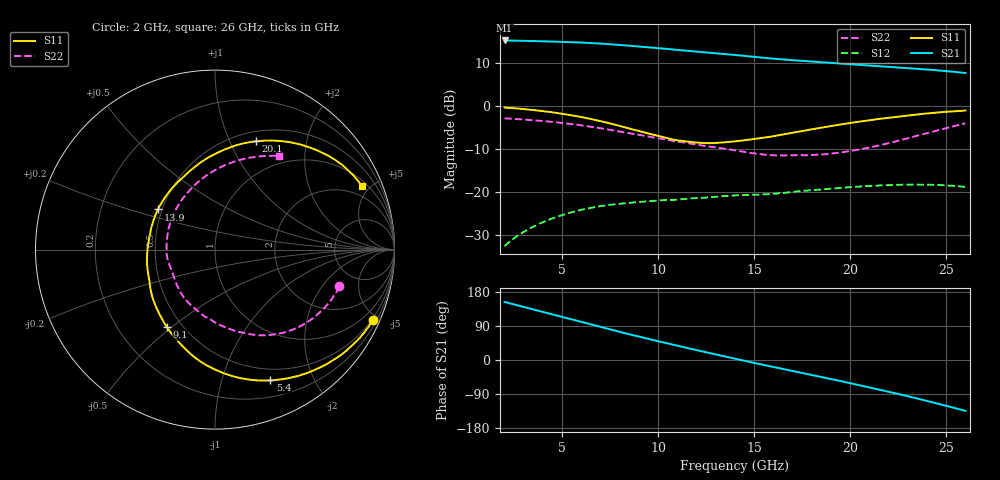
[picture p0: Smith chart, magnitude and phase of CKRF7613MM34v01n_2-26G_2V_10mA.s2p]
! CHUO DENSHI KOGYO Co.,Ltd.
! 26. October 2020
! CKRF7613MM34_RT5880
! N-channel HJ-FET
! Vds = 2 V, Id = 10 mA
# Hz S  MA  R 50
!	f	S11	S21	S12	S22
!	Hz	MAG	ANG	MAG	ANG	MAG	ANG	MAG	ANG
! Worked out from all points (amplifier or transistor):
!   241 points, 2 GHz to 26 GHz, reference 50 ohm
!   highest |S21| = 15.3 dB at 2 GHz (marker M1)
!   |S21| within 3 dB of that: start of sweep to 13.09 GHz
!   unconditionally stable (mu >= 1): 10.36 GHz to 18.29 GHz
!   at 6 GHz: K = 0.58, MSG = 19.4 dB, |S12| = -24.1 dB
!   at 14 GHz: K = 1.12, MAG = 14.2 dB, |S12| = -20.7 dB
!   at 26 GHz: K = 0.34, MSG = 13.3 dB, |S12| = -18.8 dB
!   lowest NFmin = 0.33 dB at 10 GHz
!   S11 on the Smith chart (normalised r, x): 2 GHz: 0.41, -4.64; 5.4 GHz: 0.37, -1.45; 9.1 GHz: 0.41, -0.48; 13.9 GHz: 0.47, +0.25; 20.1 GHz: 0.61, +1.25; 26 GHz: 1.29, +4.45
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2e9  0.9649 -24.1  5.826 153.1  0.02358 73.4  0.7222 -16.5
2.9e9  0.9316 -35.1  5.776 141.3  0.03353 66.7  0.7039 -24.0
3.8e9  0.8884 -46.3  5.713 129.4  0.04299 59.9  0.6787 -31.4
4.6e9  0.8436 -56.4  5.644 118.9  0.05058 54.0  0.6532 -38.2
5.4e9  0.7914 -67.0  5.57 108.4  0.05767 48.0  0.625 -45.1
6e9  0.7492 -75.2  5.504 100.5  0.06252 43.5  0.6002 -50.4
6.7e9  0.695 -85.1  5.405 91.2  0.06715 38.4  0.569 -56.6
7.4e9  0.6394 -95.4  5.29 82.0  0.07109 33.6  0.537 -62.8
8.2e9  0.5728 -107.6  5.119 71.6  0.07417 28.6  0.4986 -69.6
9.1e9  0.5075 -121.9  4.928 60.4  0.07738 24.0  0.46 -77.4
1e10  0.4521 -137.7  4.743 49.5  0.08006 19.9  0.4253 -85.3
1.07e10  0.4136 -151.1  4.587 41.0  0.08143 16.7  0.3974 -91.9
1.18e10  0.3821 -172.8  4.372 28.3  0.08501 13.0  0.3645 -102.8
1.3e10  0.3744 162.8  4.14 14.7  0.08869 9.0  0.3327 -115.8
1.39e10  0.3889 144.9  3.973 4.4  0.09162 5.4  0.3097 -127.2
1.4e10  0.3908 143.0  3.953 3.2  0.09183 4.9  0.3071 -128.4
1.56e10  0.4345 116.6  3.638 -14.1  0.09466 -0.4  0.2728 -148.6
1.8e10  0.5386 88.7  3.309 -39.3  0.1056 -8.2  0.2708 174.9
2.01e10  0.6442 69.5  3.074 -62.2  0.1153 -18.4  0.3041 139.5
2.2e10  0.7352 54.1  2.876 -83.7  0.1208 -29.4  0.372 109.0
2.4e10  0.8247 38.7  2.676 -107.9  0.1226 -43.2  0.4875 80.5
2.6e10  0.8908 23.5  2.436 -134.4  0.1151 -58.8  0.6326 55.6
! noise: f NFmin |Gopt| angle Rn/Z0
1e+10  0.33  0.391  88.2  0.09
1.05e+10  0.34  0.369  92.9  0.08
1.1e+10  0.36  0.339  100.7  0.07
1.15e+10  0.38  0.303  110.7  0.07
1.2e+10  0.39  0.27  119.5  0.06
1.25e+10  0.41  0.243  132.6  0.06
1.3e+10  0.43  0.221  145.4  0.05
1.35e+10  0.45  0.201  161.4  0.05
1.4e+10  0.48  0.194  177.7  0.05
1.5e+10  0.56  0.194  -142.8  0.06
